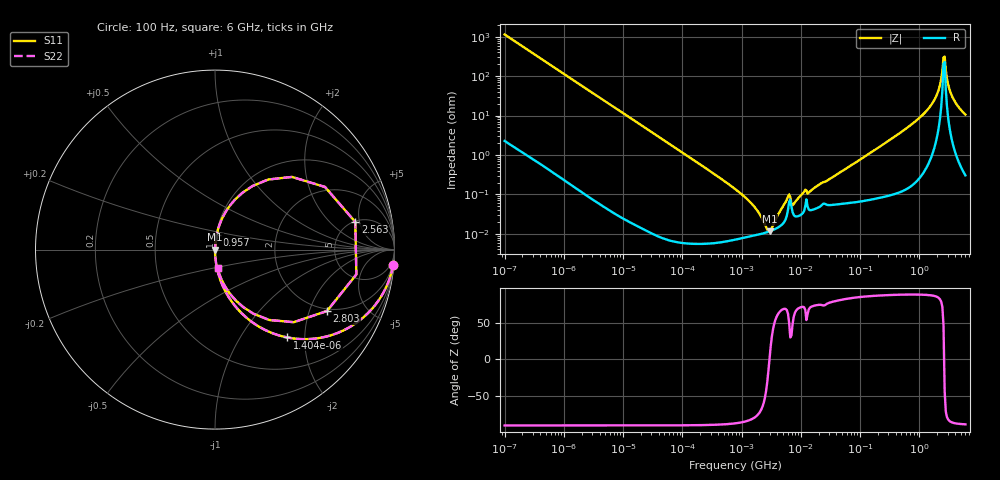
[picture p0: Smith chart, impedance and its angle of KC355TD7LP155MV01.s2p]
!Murata Part Number: KC355TD7LP155MV01
!These Parameters are Measured in Series Mode Connection
!Data Generated on Mar 13, 2026
!  o--ll--o
!Port1  Port2
!  o------o
!Operation Temp=25[degC], DC Bias Voltage=0[V]
!Freq. Start=100[Hz] Stop=6[GHz] 401[Steps]
# Hz S RI R 50
!Freq.(Hz) S11(Real) S11(Imag) S21(Real) S21(Imag) S12(Real) S12(Imag) S22(Real) S22(Imag)
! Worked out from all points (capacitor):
!   401 points, 100 Hz to 6 GHz, reference 50 ohm
!   read as one part in series: C = 1.39 uF near 109 Hz
!   lowest |Z| = 11.5 mohm at 2.968 MHz (marker M1)
!   series resonance near 2.954 MHz, so ESL is about 2.1 nH
!   S11 on the Smith chart (normalised r, x): 100 Hz: 1, -23; 1.404 kHz: 1.00, -1.64; 957 MHz: 1.00, +0.16; 2.563 GHz: 5.12, +4.31; 2.803 GHz: 1.91, -2.65; 6 GHz: 1.01, -0.21
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100  0.9923 -0.0865  0.00772 0.0865  0.00772 0.0865  0.9923 -0.0865
438  0.8724 -0.3326  0.1276 0.3326  0.1276 0.3326  0.8724 -0.3326
1404  0.402 -0.4893  0.598 0.4893  0.598 0.4893  0.402 -0.4893
2008  0.2476 -0.4307  0.7524 0.4307  0.7524 0.4307  0.2476 -0.4307
5378  0.0443 -0.2047  0.9557 0.2047  0.9557 0.2047  0.0443 -0.2047
40335  0.000902 -0.0286  0.9991 0.0286  0.9991 0.0286  0.000902 -0.0286
774597  7.26e-05 -0.00137  0.9999 0.00137  0.9999 0.00137  7.26e-05 -0.00137
1585629  8.93e-05 -0.000509  0.9999 0.000509  0.9999 0.000509  8.93e-05 -0.000509
2967816  0.000115 3.8e-06  0.9999 -3.8e-06  0.9999 -3.8e-06  0.000115 3.8e-06
6075234  0.000403 0.000772  0.9996 -0.000772  0.9996 -0.000772  0.000403 0.000772
7599586  0.0003 0.000485  0.9997 -0.000485  0.9997 -0.000485  0.0003 0.000485
1.137099e7  0.00038 0.00111  0.9996 -0.00111  0.9996 -0.00111  0.00038 0.00111
1.555665e7  0.000405 0.00127  0.9996 -0.00127  0.9996 -0.00127  0.000405 0.00127
3.124326e8  0.00149 0.0236  0.9985 -0.0236  0.9985 -0.0236  0.00149 0.0236
9.569533e8  0.00897 0.081  0.991 -0.081  0.991 -0.081  0.00897 0.081
1.873145e9  0.0889 0.2526  0.9111 -0.2526  0.9111 -0.2526  0.0889 0.2526
2.240541e9  0.2961 0.3903  0.7039 -0.3903  0.7039 -0.3903  0.2961 0.3903
2.562649e9  0.7815 0.154  0.2185 -0.154  0.2185 -0.154  0.7815 0.154
2.802721e9  0.6242 -0.3422  0.3758 0.3422  0.3758 0.3422  0.6242 -0.3422
3.065283e9  0.3026 -0.3922  0.6974 0.3922  0.6974 0.3922  0.3026 -0.3922
3.505958e9  0.1168 -0.2844  0.8832 0.2844  0.8832 0.2844  0.1168 -0.2844
6e9  0.014 -0.1038  0.986 0.1038  0.986 0.1038  0.014 -0.1038
